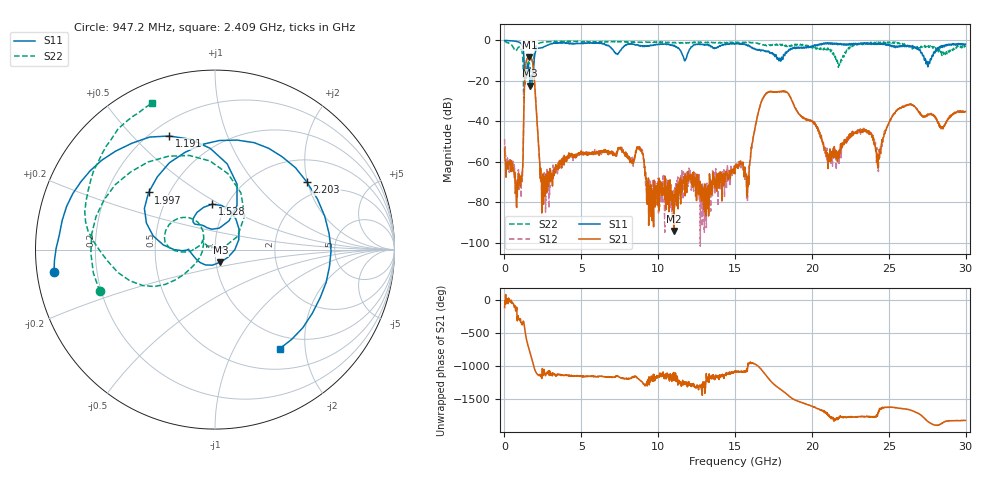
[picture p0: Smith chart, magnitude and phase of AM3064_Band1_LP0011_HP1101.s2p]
# Hz S DB R 50.0
!freq dBS11 angS11 dBS21 angS21 dBS12 angS12 dBS22 angS22
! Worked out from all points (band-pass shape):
!   1600 points, 10 MHz to 29.98 GHz, reference 50 ohm
!   highest |S21| = -8.21 dB at 1.622 GHz (marker M1); lowest = -94.2 dB at 11.01 GHz (marker M2)
!   |S21| within 3 dB of the highest: 1.398 GHz to 1.835 GHz (436.9 MHz wide, 27 % of centre)
!   lowest |S11| = -22.3 dB at 1.678 GHz (marker M3), VSWR 1.17, Z = 52.5 - j7.42 ohm
!   |S11| at or under -10 dB: 1.277 GHz to 1.93 GHz (653.5 MHz wide, 40.8 % of centre); 11.70904 GHz to 11.74829 GHz (39.25 MHz wide, 0.335 % of centre); 27.4 GHz to 27.68 GHz (281.5 MHz wide, 1.02 % of centre)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
!   |S22| runs from -29.3 to -0.3 dB; largest |S21 - S12| = 0.0058
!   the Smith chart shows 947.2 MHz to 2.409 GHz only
!   S11 on the Smith chart (normalised r, x): 947.2 MHz: 0.05, -0.07; 1.191 GHz: 0.27, +0.64; 1.528 GHz: 0.85, +0.46; 1.997 GHz: 0.39, +0.32; 2.203 GHz: 1.57, +1.98; 2.409 GHz: 0.79, -1.55
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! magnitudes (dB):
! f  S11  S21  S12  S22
! 10 MHz  -0.1  -53.4  -48.7  -0.3
! 947.2 MHz  -0.9  -66.3  -66.1  -3.3
! 1.191 GHz  -3.3  -61.9  -63.9  -9.2
! 1.528 GHz  -11.9  -8.6  -8.5  -11.0
! 1.622 GHz  -16.9  -8.2  -8.2  -11.4
! 1.678 GHz  -22.3  -8.3  -8.3  -13.7
! 1.997 GHz  -6.2  -25.2  -25.1  -4.4
! 2.203 GHz  -3.9  -50.2  -49.3  -1.7
! 2.409 GHz  -3.6  -67.9  -67.4  -1.0
! 5.015 GHz  -1.3  -56.2  -56.0  -0.8
! 8.782 GHz  -2.6  -52.5  -53.1  -0.9
! 10 GHz  -2.0  -74.2  -68.2  -0.9
! 11.01 GHz  -2.7  -94.2  -73.7  -1.2
! 15 GHz  -1.7  -66.0  -61.9  -1.3
! 15.79 GHz  -2.5  -77.3  -72.4  -1.1
! 17.14 GHz  -5.7  -25.7  -25.6  -2.6
! 19.99 GHz  -3.3  -39.9  -40.0  -3.4
! 21.19 GHz  -1.9  -59.5  -56.2  -5.0
! 23.46 GHz  -1.6  -44.8  -44.5  -1.4
! 24.34 GHz  -2.0  -58.7  -63.0  -1.2
! 25 GHz  -2.0  -41.1  -41.0  -1.1
! 29.98 GHz  -1.9  -35.1  -35.3  -3.3
